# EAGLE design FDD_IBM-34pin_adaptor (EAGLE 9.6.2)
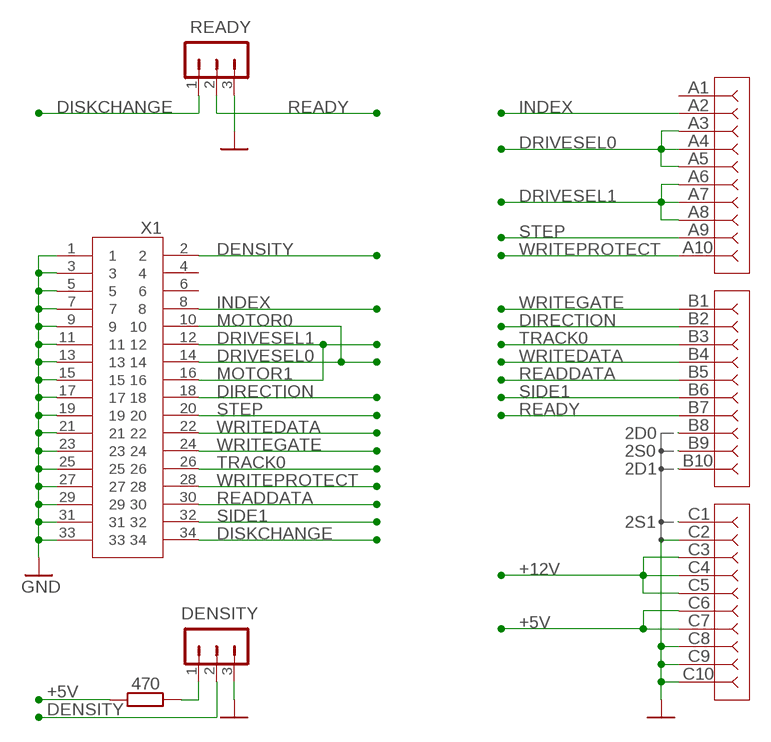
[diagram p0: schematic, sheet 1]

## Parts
DENSITY  JP3S  [JP3S]
R1  470  R-EU_0207/7  [0207/7]
READY  JP3S  [JP3S]
U$2  FDD-30PIN  [FDD-30PIN]
X1  057-034-B  [057-034-1]

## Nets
2D0: U$2.B8
2D1: U$2.B10
2S0: U$2.B9
2S1: U$2.C1
+5V: R1.1 U$2.C6 U$2.C7
+12V: U$2.C3 U$2.C4 U$2.C5
DENSITY: DENSITY.2 X1.2
DIRECTION: U$2.B2 X1.18
DISKCHANGE: READY.1 X1.34
DRIVESEL0: U$2.A3 U$2.A4 U$2.A5 X1.10 X1.14
DRIVESEL1: U$2.A6 U$2.A7 U$2.A8 X1.12 X1.16
GND: DENSITY.3 READY.3 U$2.C2 U$2.C8 U$2.C9 U$2.C10 X1.1 X1.3 X1.5 X1.7 X1.9 X1.11 X1.13 X1.15 X1.17 X1.19 X1.21 X1.23 X1.25 X1.27 X1.29 X1.31 X1.33
INDEX: U$2.A2 X1.8
N$1: DENSITY.1 R1.2
READDATA: U$2.B5 X1.30
READY: READY.2 U$2.B7
SIDE1: U$2.B6 X1.32
STEP: U$2.A9 X1.20
TRACK0: U$2.B3 X1.26
WRITEDATA: U$2.B4 X1.22
WRITEGATE: U$2.B1 X1.24
WRITEPROTECT: U$2.A10 X1.28
Unconnected: U$2.A1 X1.4 X1.6

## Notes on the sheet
- MOTOR0
- MOTOR1

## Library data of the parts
DENSITY READY = jumpers_lib:JP3S
R1 = rcl:R-EU_: RESISTOR, European symbol; SPICEPREFIX: R
U$2 = AGAT_Slot_Connector:FDD-30PIN
X1 = con-panduit:057-034-: CONNECTOR 34-pin series 057 contact pc board low profile headers

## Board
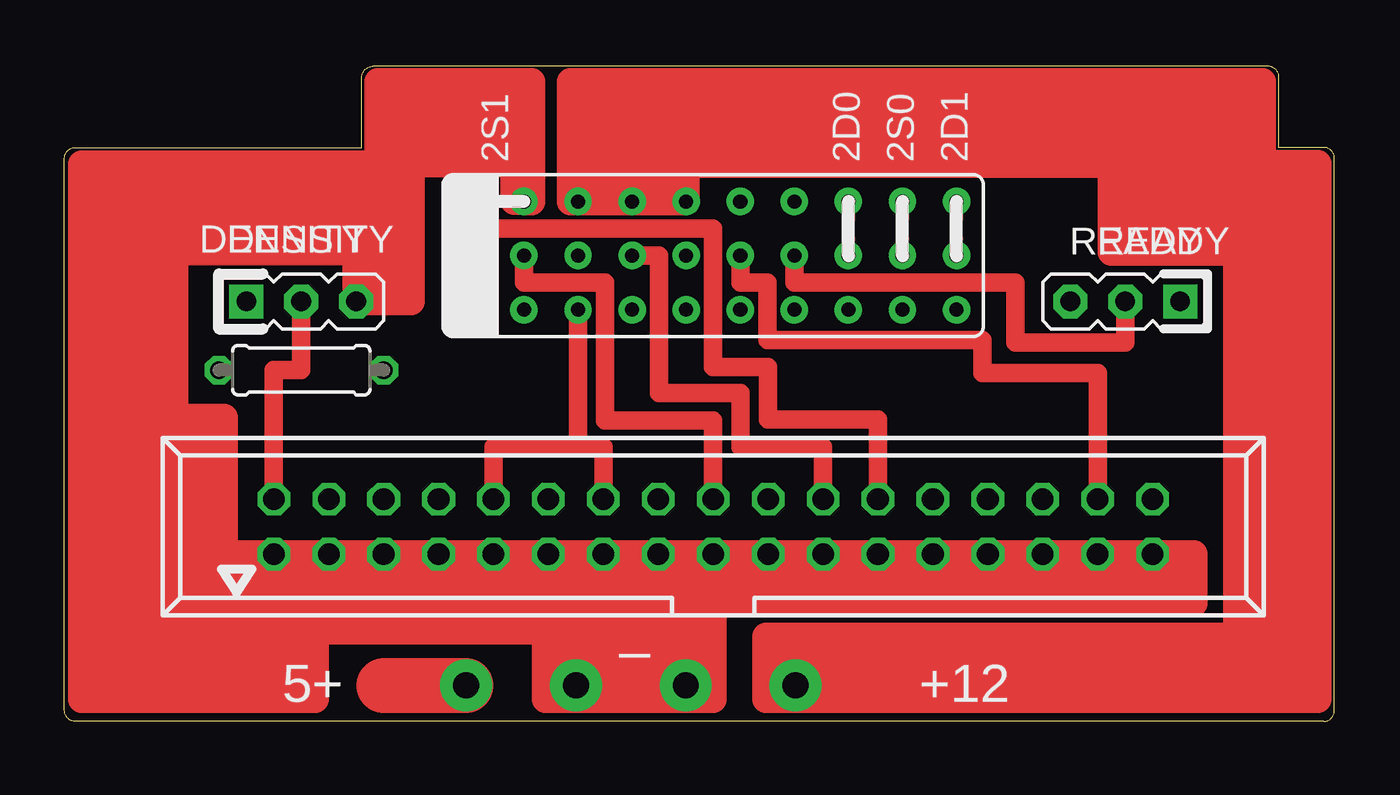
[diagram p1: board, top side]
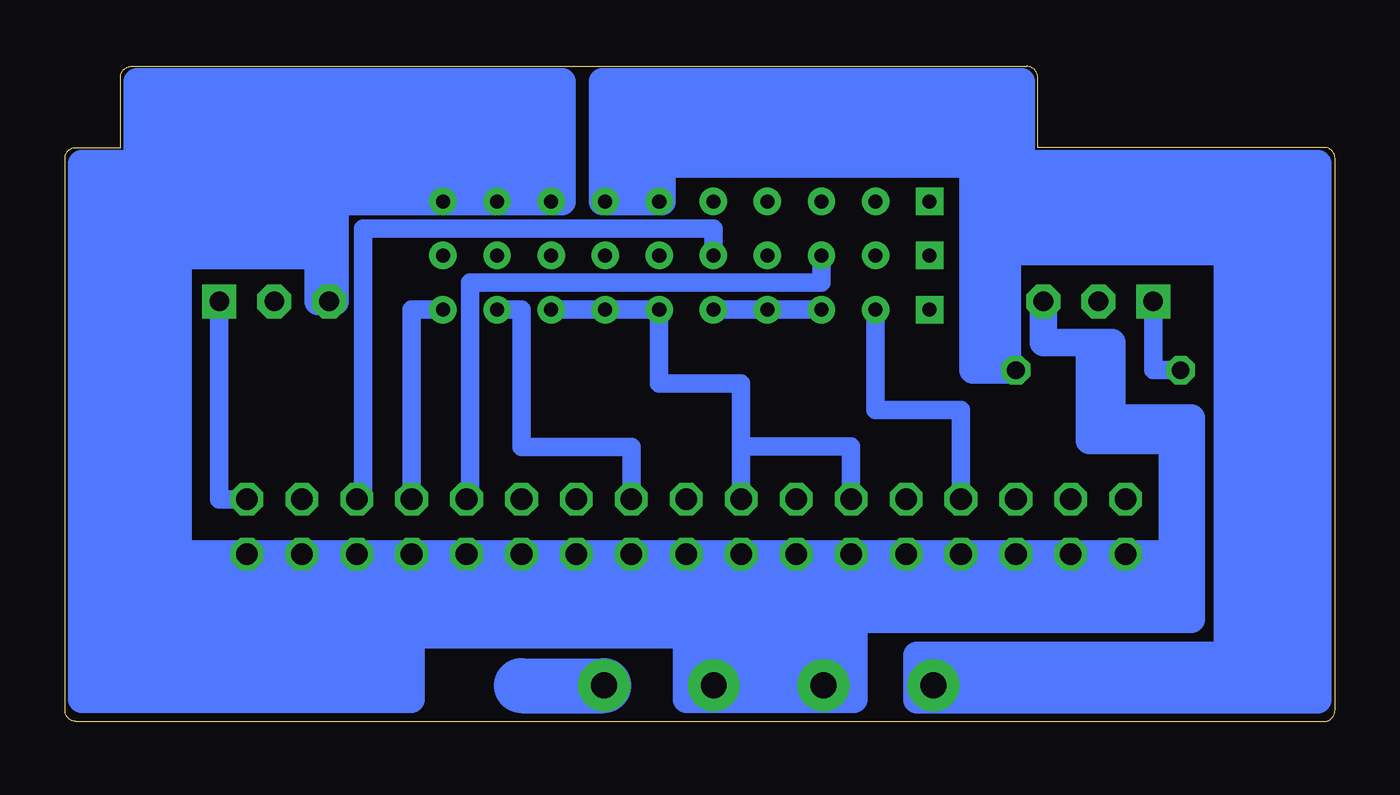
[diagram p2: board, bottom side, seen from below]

Size 58.73 x 30.29 mm. Coordinates in mm from the lower left corner, seen from the top.
Outline: 58.23,0 0.5,0 arc-90 0,0.5 0,26.04 arc-90 0.5,26.54 13.75,26.54 13.75,29.79 arc-90 14.25,30.29 55.66,30.29 arc-90 56.16,29.79 56.16,26.54 58.23,26.54 arc-90 58.73,26.04 58.73,0.5 arc-90 58.23,0
Copper layers (1*16): Top 0.035mm / dielectric 1.5mm / Bottom 0.035mm
Design rules "default *": minimum track width 6mil, minimum drill 0.35mm, track to track 6mil, track to pad 6mil, pad to pad 6mil, via to via 6mil, smd to smd 6mil, copper to edge 0mil, drill to drill 6mil, minimum pad ring 10mil, minimum via ring 8mil, stop-mask expansion 0mil, vias tented up to drill 0mil, thermal gap 10mil

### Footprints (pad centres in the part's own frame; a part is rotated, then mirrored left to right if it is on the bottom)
JP3S = drill 0.914 pad 1.57 square: 1 -2.54,0 | drill 0.914 pad 1.57 octagon: 2 0,0; 3 2.54,0
0207/7 = drill 0.813 octagon: 1 -3.81,0; 2 3.81,0
FDD-30PIN = drill 0.65 pad 1.27 square: A1 -11.25,-2.5; B1 -11.25,0; C1 -11.25,2.5 | drill 0.65 pad 1.27: A2 -8.75,-2.5; A3 -6.25,-2.5; A4 -3.75,-2.5; A5 -1.25,-2.5; A6 1.25,-2.5; A7 3.75,-2.5; A8 6.25,-2.5; A9 8.75,-2.5; A10 11.25,-2.5; B2 -8.75,0; B3 -6.25,0; B4 -3.75,0; B5 -1.25,0; B6 1.25,0; B7 3.75,0; B8 6.25,0; B9 8.75,0; B10 11.25,0; C2 -8.75,2.5; C3 -6.25,2.5; C4 -3.75,2.5; C5 -1.25,2.5; C6 1.25,2.5; C7 3.75,2.5; C8 6.25,2.5; C9 8.75,2.5; C10 11.25,2.5
057-034-1 = drill 1 octagon: 1 -20.32,-1.27; 2 -20.32,1.27; 3 -17.78,-1.27; 4 -17.78,1.27; 5 -15.24,-1.27; 6 -15.24,1.27; 7 -12.7,-1.27; 8 -12.7,1.27; 9 -10.16,-1.27; 10 -10.16,1.27; 11 -7.62,-1.27; 12 -7.62,1.27; 13 -5.08,-1.27; 14 -5.08,1.27; 15 -2.54,-1.27; 16 -2.54,1.27; 17 0,-1.27; 18 0,1.27; 19 2.54,-1.27; 20 2.54,1.27; 21 5.08,-1.27; 22 5.08,1.27; 23 7.62,-1.27; 24 7.62,1.27; 25 10.16,-1.27; 26 10.16,1.27; 27 12.7,-1.27; 28 12.7,1.27; 29 15.24,-1.27; 30 15.24,1.27; 31 17.78,-1.27; 32 17.78,1.27; 33 20.32,-1.27; 34 20.32,1.27

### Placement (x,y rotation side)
DENSITY  10.95,19.42 0 top
R1  10.95,16.24 180 top
READY  49.05,19.42 180 top
U$2  30,21.54 0 top
X1  30,9 0 top

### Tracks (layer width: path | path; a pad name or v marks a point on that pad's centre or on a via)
2D0
  Top 0.61: 36.26,22.33 U$2.B8
2D1
  Top 0.61: 41.26,22.33 U$2.B10
2S0
  Top 0.61: 38.76,22.33 U$2.B9
2S1
  Top 0.61: 19.54,24.04 U$2.C1
+5V  (via drill 1.2 pad 2.4)
  Bottom 1.27: 31.93,24.04 U$2.C6 31.12,24.04 31.12,25.78 16.75,25.78 16.75,21.73 | 31.93,24.04 32.83,24.04 | 32.83,24.04 U$2.C7 33.88,24.04 33.88,29.6 14.5,29.6 14.5,28.59 | 2.72,24.97 2.72,23.7 2.97,23.7 | 3.99,21.73 3.99,3.06 4.98,3.06 | 3.99,21.73 3.99,22.73 | 3.99,22.73 3.99,24.97 | 2.72,24.97 2.72,25.79 | 3.99,24.97 2.72,24.97 | 2.97,23.7 10.09,23.7 | 10.09,23.7 10.09,23.87 | 10.09,23.87 10.09,24.85 | 10.09,24.85 10.09,24.97 | 10.09,24.97 10.09,25.79 | 3.99,24.97 6.53,24.97 | 6.53,24.97 10.09,24.97 | 2.72,25.79 6.53,25.79 | 6.53,25.79 10.09,25.79 | 31.93,26.66 31.93,24.04 | 32.83,24.04 32.83,28.59 14.5,28.59 | 6.53,25.79 6.53,24.97 | 1.83,25.79 2.72,25.79 | 1.83,25.79 0.79,25.79 0.79,1 1.83,1 | 10.09,23.7 10.09,22.73 | 14.5,27.67 14.5,26.66 | 14.5,27.67 14.5,28.59 | 14.5,27.67 31.93,27.67 31.93,26.66 | 31.93,26.66 15.64,26.66 | 15.64,26.66 14.5,26.66 | 16.75,21.73 15.64,21.73 | 10.09,22.73 4.98,22.73 | 4.98,22.73 3.99,22.73 | 15.64,26.66 15.64,21.73 | 14.62,24.85 14.62,25.79 14.5,25.79 | 14.62,24.85 14.62,23.87 | 14.62,23.87 14.62,22.73 | 14.62,22.73 14.62,21.73 | 10.09,24.85 14.62,24.85 | 14.62,22.73 10.09,22.73 | 14.62,23.87 10.09,23.87 | 10.09,25.79 14.5,25.79 | 14.5,25.79 14.5,26.66 | 14.62,21.73 15.14,21.73 15.14,18.66 | 16.75,18.66 16.75,21.73 | 14.62,21.73 3.99,21.73 | 15.14,18.66 15.14,16.24 R1.1 16.03,16.24 | 17.82,3.06 17.96,2.81 v18.57,1.66 18.32,1.92 2.97,1.92 2.97,23.7 | 17.82,3.06 4.98,3.06 | 1.83,1 19.33,1 19.33,3.06 17.82,3.06 | 1.83,25.79 1.83,1 | 15.64,21.73 15.64,19.42 | 15.64,19.42 15.64,18.66 | 15.64,18.66 16.75,18.66 | 15.14,18.66 15.64,18.66 | 4.98,22.73 4.98,3.06 | 16.03,16.24 16.75,16.24 16.75,18.66 | 15.64,19.42 16.03,19.42 16.03,16.24
+12V  (via drill 1.2 pad 2.4)
  Top 1.27: 27.87,24.04 U$2.C5 28.75,25.77 | 27.87,24.04 26.85,24.04 | 26.85,24.04 U$2.C4 | U$2.C4 25.33,24.04 | 25.33,24.04 24.56,24.04 | 24.56,24.04 U$2.C3 | 32.44,3.06 32.44,1.03 57.95,1.03 57.95,1.92 | 28.75,26.66 28.75,25.77 | 32.44,3.06 55.4,3.06 | 55.4,3.06 55.91,3.06 | 57.03,25.79 57.03,3.06 55.91,3.06 | 24.56,24.04 24.56,27.43 | 24.56,27.43 25.33,27.43 | 25.33,24.04 25.33,27.43 | 26.85,24.04 26.85,27.43 | 26.85,27.43 26.25,27.43 | 26.25,27.43 25.33,27.43 | 23.75,27.43 24.56,27.43 | U$2.C3 23.75,27.43 | 26.85,27.43 27.87,27.43 | 27.87,27.43 27.87,27.68 53.88,27.68 | 27.87,27.43 27.87,24.04 | 23.75,28.57 23.75,27.43 | 23.75,28.57 23.75,29.58 | 53.88,27.68 55.4,27.68 | 57.95,1.92 33.45,1.92 v33.81,1.66 | 32.44,3.06 32.44,3.93 54.22,3.93 54.22,21.71 | U$2.C4 26.25,27.43 | 55.4,27.68 55.4,3.06 | 53.88,27.68 53.88,26.66 | 54.26,25.77 54.26,26.66 53.88,26.66 | 54.26,25.77 54.26,24.63 54.13,24.63 | 54.13,24.63 54.13,23.49 | 54.26,22.47 54.26,23.49 54.13,23.49 | 28.75,25.77 48.41,25.77 | 48.41,25.77 49.05,25.77 | 49.05,25.77 54.26,25.77 | 54.22,21.71 54.51,21.71 54.51,22.47 54.26,22.47 | 54.22,21.71 48.41,21.71 48.41,22.47 | 48.41,22.47 48.41,25.77 | 49.05,24.63 49.05,23.49 54.13,23.49 | 49.05,24.63 49.05,25.77 | 54.13,24.63 49.05,24.63 | 54.26,22.47 48.41,22.47 | U$2.C3 23.4,24.05 23.4,29.58 23.75,29.58 | 28.75,26.66 28.75,26.81 | 53.88,26.66 28.75,26.66 | 57.03,25.79 55.91,25.79 55.91,3.06 | 57.03,25.79 57.95,25.79 57.95,1.92 | 55.4,28.57 55.4,27.68 | 23.75,28.57 55.4,28.57 | 55.4,28.57 55.4,29.58 23.75,29.58
DENSITY
  Top 0.86: DENSITY.2 10.95,16.25 9.68,16.25 X1.2
DIRECTION
  Top 0.86: X1.18 30,13.91 25,13.91 25,20.3 21.25,20.3 U$2.B2
DISKCHANGE
  Bottom 0.86: X1.34 51.59,10.27 READY.1
DRIVESEL0
  Top 0.86: X1.14 24.92,12.69 23.75,12.69 | 23.75,12.69 U$2.A3 | 23.75,12.69 19.84,12.69 X1.10
  Bottom 0.86: U$2.A3 U$2.A4 U$2.A5
DRIVESEL1
  Bottom 0.86: X1.12 22.38,12.71 27.46,12.71 | U$2.A8 U$2.A7 U$2.A6 31.25,15.63 27.46,15.63 27.46,12.71 | X1.16 27.46,12.71
GND  (via drill 1.2 pad 2.4)
  Top 0.61: 41.26,23.25 U$2.C10 | 38.76,23.25 U$2.C9 | 36.26,23.25 U$2.C8 | 21.23,24.06 U$2.C2 20.46,24.04 20.45,24.04
  Top 1.27: X1.33 X1.31 X1.29 X1.27 X1.25 X1.23 X1.21 X1.19 X1.17 X1.15 X1.13 X1.11 X1.9 X1.7 | X1.7 17.3,6.72 | 17.3,6.72 17.3,6.52 | 17.3,6.52 17.3,5.72 | 17.3,6.72 50.32,6.72 | 50.32,6.72 51.08,6.72 51.08,5.45 | 50.32,6.72 X1.33 | 51.08,5.45 30,5.45 | 9.68,4.18 9.68,5.2 0.79,5.2 | 11.59,4.18 9.68,4.18 | 7.39,7.73 X1.1 X1.3 X1.5 | 7.39,7.73 6.2,7.73 6.2,13.07 5.22,13.07 | 3.96,21.73 3.96,13.07 | 3.96,21.73 3.96,21.96 | 4.6,22.43 4.6,21.96 3.96,21.96 | 4.6,22.43 4.6,23.23 | 4.6,23.23 4.6,24.5 | 4.6,24.5 4.6,25.77 | 0.79,4.18 3.71,4.18 | 3.71,4.18 9.68,4.18 | 2.7,25.77 1.68,25.77 | 1.68,25.77 0.79,25.77 0.79,6.72 | 0.79,5.2 0.79,6.72 | 0.79,5.2 0.79,4.18 | 0.79,1.64 0.79,1.01 3.71,1.01 | 0.79,4.18 0.79,2.91 | 3.71,4.18 3.71,2.91 | 3.71,2.91 3.71,2.02 | 3.71,2.02 3.71,1.64 | 3.71,1.64 3.71,1.01 | 0.79,2.91 3.71,2.91 | 0.79,2.91 0.79,1.64 | 0.79,1.64 3.71,1.64 | 5.27,7.18 5.08,7.18 5.08,13.07 | 5.27,7.18 9.74,7.18 9.74,6.51 | 1.68,6.72 2.7,6.72 | 1.68,6.72 1.53,6.72 | 1.68,6.72 1.68,25.77 | 2.7,6.72 2.7,6.43 3.33,6.43 | 2.7,6.72 2.7,9.26 | 2.7,9.26 2.7,25.77 | 51.08,5.45 52.23,5.45 52.23,7.73 X1.33 | 2.7,25.77 3.41,25.77 | 3.41,25.77 4.6,25.77 | 16.03,24.04 16.03,23.23 | 16.03,23.23 16.03,21.96 | 16.03,21.96 16.03,20.69 | 16.03,20.69 16.03,19.42 DENSITY.3 13.49,20.69 | 21.25,29.58 U$2.C2 21.59,24.04 21.59,29.58 21.25,29.58 | 21.25,29.58 20.11,29.58 | 20.11,29.58 19.22,29.58 | 18.57,29.58 17.19,29.58 | 17.19,29.58 16.03,29.58 | 16.03,29.58 15.14,29.58 | 4.6,25.77 14.51,25.77 14.51,29.58 15.14,29.58 | 4.6,22.43 5.11,22.43 | 5.11,22.43 12.22,22.43 12.22,21.96 16.03,21.96 | 4.6,23.23 16.03,23.23 | 4.6,24.5 15.14,24.5 | 15.14,24.5 15.14,29.58 | 16.03,24.04 15.14,24.04 15.14,24.5
  Top 1.27: 16.03,24.04 16.03,25.79 | 16.03,25.79 16.03,29.58 | 19.22,25.79 19.22,29.58 | 20.11,25.79 20.11,29.58 | 19.22,29.58 18.19,29.58 18.19,26.58 | 13.49,20.69 13.49,21.73 3.96,21.73 | 13.49,20.69 16.03,20.69 | 5.27,6.72 5.27,7.18 | 5.08,13.07 3.96,13.07 | 5.22,13.07 5.22,14.07 7.39,14.07 7.39,7.73 | 5.22,13.07 5.11,13.07 5.11,22.43 | 3.71,1.01 11.59,1.01 11.59,2.02 | 11.59,2.02 11.59,2.91 | 11.59,2.91 11.59,4.18 | 22.25,4.18 30,4.18 | 30,4.18 30,5.45 | 3.71,2.91 11.59,2.91 | 11.59,2.02 3.71,2.02 | 30,4.18 30,2.91 | 30,2.91 30,1.64 | 30,1.64 30,1.01 22.25,1.01 22.25,1.64 | 22.25,1.64 22.25,2.91 | 22.25,2.91 22.25,4.18 | 22.25,1.64 30,1.64 | 30,2.91 22.25,2.91 | 5.59,13.07 5.08,13.07 | 20.11,25.79 20.79,25.79 20.79,24.06 21.23,24.06 | 17.19,25.79 19.22,25.79 | 19.22,25.79 20.11,25.79 | 17.19,29.58 17.19,25.79 | 17.19,25.79 16.03,25.79 | X1.5 X1.7 | 11.59,4.18 22.25,4.18 | 14.76,6.52 17.3,6.52 | 3.96,21.96 3.41,22.52 3.41,25.77 | 0.79,6.72 1.53,6.72 | 1.53,6.72 1.53,5.45 30,5.45 | 3.33,6.43 3.96,6.43 | 3.96,6.43 9.74,6.43 9.74,6.51 | 9.74,6.51 14.76,6.51 X1.5 | 2.7,9.26 3.33,9.26 3.33,6.43 | 3.96,13.07 3.96,6.43
  Bottom 1.27: X1.7 17.3,6.74 | 17.3,6.74 17.3,5.73 | X1.7 X1.9 | X1.9 X1.11 X1.13 X1.15 X1.17 X1.19 X1.21 X1.23 X1.25 X1.27 X1.29 X1.31 X1.33 54.66,7.73 | 54.66,7.73 55.6,7.73 | U$2.C10 U$2.C9 U$2.C8 35.74,24.04 35.74,25.29 | 35.74,25.79 35.74,26.67 | 35.74,25.29 35.74,25.79 | 41.38,24.79 41.38,24.04 U$2.C10 | 41.25,25.29 41.25,25.79 | 35.74,25.29 41.25,25.29 | 41.25,25.29 41.38,25.29 41.38,24.79 | 35.74,25.79 41.25,25.79 | 17.3,5.73 17.3,4.71 | 12.22,5.73 12.22,4.71 | X1.9 19.84,6.74 | 19.84,6.74 17.3,6.74 | 19.84,6.74 53.5,6.74 53.5,21.54 | 53.86,5.73 17.3,5.73 | 53.86,5.73 56.65,5.73 | 53.86,5.73 53.86,6.74 56.77,6.74 | 17.3,4.71 22.25,4.71 | 22.25,4.71 22.63,4.71 | 22.63,4.71 56.77,4.71 | 56.77,4.71 57.97,4.71 | 12.22,5.73 6.66,5.73 | 12.22,4.71 6.66,4.71 6.66,5.73 | 35.74,28.54 35.74,29.59 55.4,29.59 55.4,28.54 | 35.74,28.54 35.74,27.67 | 35.74,27.67 35.74,26.67 | 42.73,4 30,4 | 30,4 28.63,4 28.63,3.55 | 53.5,24.04 54.66,24.04 | 53.5,21.54 53.5,22.41 | 53.5,22.41 53.5,23.36 | 53.5,23.36 53.5,24.04 | 55.6,25.79 55.6,7.73 | 41.25,25.79 55.4,25.79 | 41.38,24.79 54.73,24.79 54.73,24.04 54.66,24.04 | DENSITY.3 13.49,17.52 11.37,17.52 | 11.37,17.52 11.37,13 7.52,13 7.52,7.73 X1.1 X1.3 X1.5 X1.7 | 11.37,17.52 10.32,17.52 10.32,14.04 6.66,14.04 6.66,6.74 | 6.66,5.73 6.66,6.74 | 22.25,2.28 22.25,1.01 23.65,1.01 | 22.25,2.28 22.25,4.71 | 23.65,1.01 v23.65,1.66 23.02,1.66 23.02,3.55 | 28.63,2.28 28.63,1.66 v28.73,1.66 | 22.63,4.71 22.63,3.55 23.02,3.55 | 23.02,3.55 28.63,3.55 | 28.63,3.55 28.88,3.55 28.88,2.28 28.63,2.28 | 22.25,2.28 28.63,2.28 | 23.65,1.01 30,1.01 30,4 | 42.73,4 42.73,1.03 57.97,1.03 57.97,2 | 55.6,7.73 56.75,7.73 | 56.75,7.73 56.78,7.73 56.78,6.74 56.77,6.74
  Bottom 1.27: 56.77,6.74 56.77,4.71 | 46.51,21.54 46.23,21.54 | 46.51,21.54 READY.3 | 46.51,21.54 47.03,21.54 | 47.03,21.54 53.5,21.54 | 54.66,24.04 54.66,7.73 | 55.4,25.79 55.6,25.79 | 55.6,25.79 56.75,25.79 | 56.75,25.79 56.75,7.73 | 56.75,25.79 57.97,25.79 57.97,4.71 | 55.4,27.67 55.4,26.67 | 55.4,26.67 55.4,25.79 | 35.74,28.54 55.4,28.54 | 55.4,27.67 55.4,28.54 | 35.74,27.67 55.4,27.67 | 35.74,26.67 55.4,26.67 | READY.3 46.23,19.42 46.23,21.54 | 57.97,4.71 57.97,4 | 57.97,4 42.73,4 | 57.97,4 57.97,3 | 57.97,3 42.75,3 42.75,2 57.97,2 | 57.97,3 57.97,2 | U$2.C10 53.5,24.04 | 46.23,21.54 46.23,22.41 | 46.23,22.41 46.23,23.36 53.5,23.36 | 53.5,22.41 46.23,22.41 | READY.3 47.03,19.42 47.03,21.54 | 17.3,5.73 12.22,5.73 | 12.22,4.71 17.3,4.71 | 17.3,6.74 6.66,6.74
INDEX
  Bottom 0.86: U$2.A2 21.25,14.4 17.3,14.4 X1.8
N$1
  Bottom 0.86: DENSITY.1 8.41,16.24 R1.2
N$2
  Top 2.54: 18.57,1.64 14.76,1.64
N$9
  Bottom 2.54: 37.62,1.64 33.81,1.64
READDATA
  Bottom 0.86: U$2.B5 28.75,22.79 44.94,22.79 44.94,10.27 X1.30
READY
  Top 0.86: U$2.B7 33.75,20.29 43.97,20.29 43.97,17.52 49.05,17.52 READY.2
SIDE1
  Top 0.86: X1.32 47.78,16.12 42.45,16.12 42.45,17.65 32.5,17.65 32.5,20.31 31.25,20.31 U$2.B6
STEP
  Bottom 0.86: U$2.A9 37.61,19.04 37.61,12.69 32.54,12.69 X1.20
TRACK0
  Bottom 0.61: X1.26 40,10.43
  Bottom 0.86: U$2.B3 23.75,20.29 40,20.29 40,10.43
WRITEDATA
  Top 0.86: X1.22 35.08,12.69 31.27,12.69 31.27,15.18 27.5,15.18 27.5,21.54 U$2.B4
WRITEGATE
  Top 0.86: X1.24 37.62,13.96 32.54,13.96 32.54,16.4 30,16.4 30,22.78 18.75,22.78 U$2.B1
WRITEPROTECT
  Bottom 0.86: X1.28 42.7,19.04 U$2.A10

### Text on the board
tPlace: 2S1 | 2D0 | 2S0 | 2D1 | _ | 5+ | +12
_tNames: DENSITY | READY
